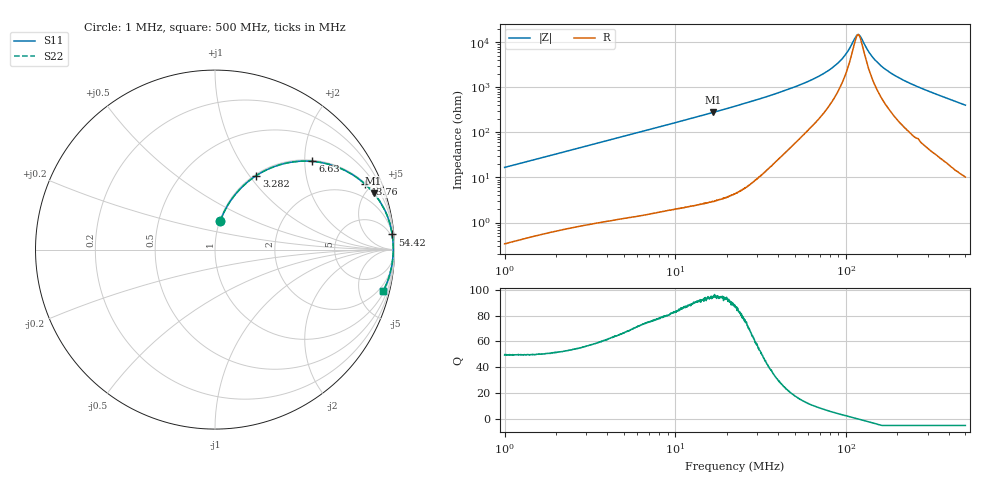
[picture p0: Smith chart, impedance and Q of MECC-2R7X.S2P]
!s-Parameter Generated by FASTRON Sdn. Bhd.
!FASTRON P/N : MECC-2R7X
!Keysight Technologies,E4991B,MY54100416,A.01.15
!Date: Wed Mar 18 10:08:16 2026
!Version  : Rev00 Wed Mar 18 10:08:16 2026
!Data & Calibration Information:
!PortZ  Port1:50+j0  Port2:50+j0
!When reading, reference impedance value at option line is always used.
! Remarks : This data is being provided solely for informational purposes.
!Freq	S11	S21	S12	S22
# Hz S dB R 50
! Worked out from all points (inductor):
!   1601 points, 1 MHz to 500 MHz, reference 50 ohm
!   read as one part in series: L = 2.66 uH near 1.032 MHz
!   highest Q = 95 at 16.71 MHz (marker M1), where L = 2.66 uH
!   self-resonance near 117.7 MHz
!   S11 on the Smith chart (normalised r, x): 1 MHz: 1.01, +0.33; 3.282 MHz: 1.02, +1.08; 6.63 MHz: 1.03, +2.18; 13.76 MHz: 1.05, +4.56; 54.42 MHz: 3, +23; 500 MHz: 1.20, -8.05
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1000000  -15.67 79.4  -0.15 -9.5  -0.15 -9.5  -15.67 79.4
1769978  -11.03 72.6  -0.41 -16.3  -0.41 -16.3  -11.03 72.6
2820919  -7.54 64.2  -0.91 -24.8  -0.91 -24.8  -7.54 64.2
3282298  -6.51 60.8  -1.18 -28.2  -1.18 -28.2  -6.51 60.8
6629778  -2.71 42.2  -3.46 -47.0  -3.46 -47.0  -2.71 42.2
7957584  -2.05 37.1  -4.39 -52.1  -4.39 -52.1  -2.05 37.1
1.37603e7  -0.80 23.6  -7.96 -65.8  -7.96 -65.8  -0.80 23.6
1.670978e7  -0.55 19.6  -9.47 -69.8  -9.47 -69.8  -0.55 19.6
2.236068e7  -0.31 14.7  -11.93 -74.7  -11.93 -74.7  -0.31 14.7
5.442207e7  -0.08 4.9  -21.36 -81.3  -21.36 -81.3  -0.08 4.9
6.307767e7  -0.07 3.8  -23.47 -80.9  -23.47 -80.9  -0.07 3.8
7.689627e7  -0.07 2.5  -27.00 -79.1  -27.00 -79.1  -0.07 2.5
9.01709e7  -0.06 1.6  -31.04 -74.7  -31.04 -74.7  -0.06 1.6
9.97527e7  -0.06 1.0  -34.84 -67.5  -34.84 -67.5  -0.06 1.0
1.133942e8  -0.06 0.2  -42.25 -29.4  -42.25 -29.4  -0.06 0.2
1.174283e8  -0.06 0.0  -43.46 -2.5  -43.46 -2.5  -0.06 0.0
1.216058e8  -0.06 -0.2  -42.49 26.2  -42.49 26.2  -0.06 -0.2
1.350515e8  -0.06 -0.8  -36.15 63.8  -36.15 63.8  -0.06 -0.8
1.453951e8  -0.06 -1.2  -32.83 71.7  -32.83 71.7  -0.06 -1.2
1.77937e8  -0.07 -2.5  -27.02 79.0  -27.02 79.0  -0.07 -2.5
2.553547e8  -0.09 -5.2  -20.76 80.7  -20.76 80.7  -0.09 -5.2
5e8  -0.31 -13.9  -12.41 74.7  -12.41 74.7  -0.31 -13.9
